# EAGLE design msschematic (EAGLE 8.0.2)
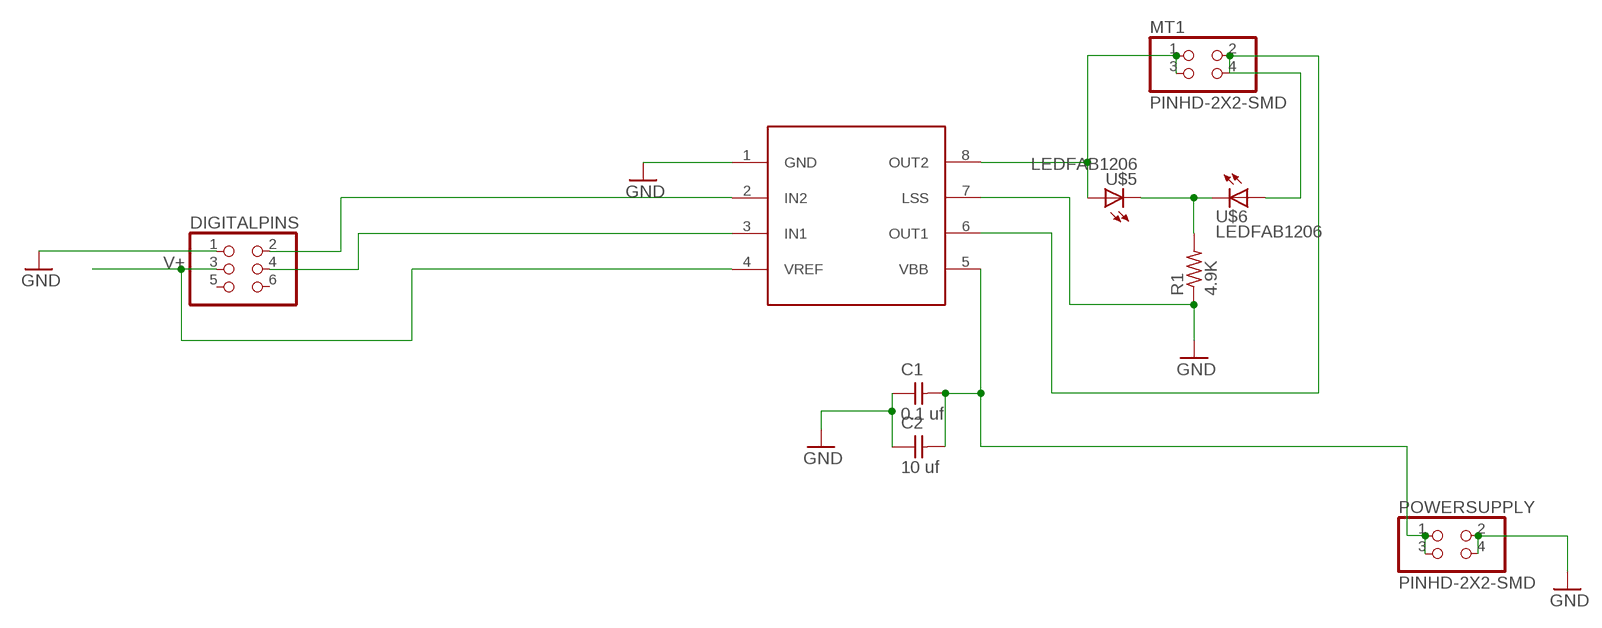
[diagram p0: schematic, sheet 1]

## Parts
C1  0.1 uf  CAP-UNPOLARIZEDFAB  [C1206FAB]
C2  10 uf  CAP-UNPOLARIZEDFAB  [C1206FAB]
DIGITALPINS  PINHD-2X3-SMD  [2X03SMD]
MT1  PINHD-2X2-SMD  [2X02SMD]
POWERSUPPLY  PINHD-2X2-SMD  [2X02SMD]
R1  4.9K  RES-US1206FAB  [R1206FAB]
U$1  A4953-H-BRIDGE-MOTOR-DRIVER  [SOIC8]
U$5  LEDFAB1206  [LED1206FAB]
U$6  LEDFAB1206  [LED1206FAB]

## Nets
GND: C1.1 C2.1 DIGITALPINS.1 POWERSUPPLY.2 POWERSUPPLY.4 R1.1 U$1.1(GND) U$1.7(LSS)
N$1: R1.2 U$5.2(C) U$6.2(C)
N$3: MT1.1 MT1.3 U$1.8(OUT2) U$5.1(A)
N$4: MT1.2 MT1.4 U$1.6(OUT1) U$6.1(A)
N$11: C1.2 C2.2 POWERSUPPLY.1 POWERSUPPLY.3 U$1.5(VBB)
N$16: DIGITALPINS.4 U$1.3(IN1)
N$17: DIGITALPINS.2 U$1.2(IN2)
V+: DIGITALPINS.3 U$1.4(VREF)
Unconnected: DIGITALPINS.5 DIGITALPINS.6

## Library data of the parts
C1 C2 = fab:CAP-UNPOLARIZED
DIGITALPINS = fab:PINHD-2X3-SMD: PIN HEADER
MT1 POWERSUPPLY = fab:PINHD-2X2-SMD
R1 = fab:RES-US: Resistor (US Symbol)
U$1 = fab:A4953-H-BRIDGE-MOTOR-DRIVER
U$5 U$6 = fab:LED: LED

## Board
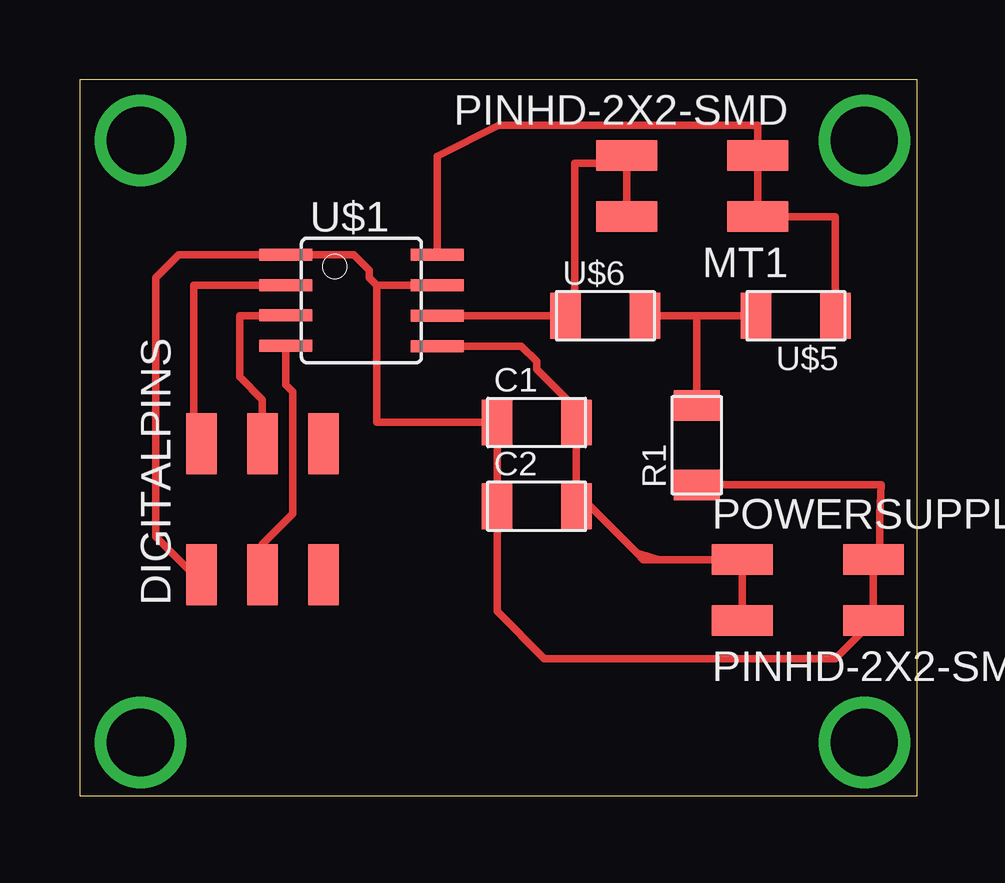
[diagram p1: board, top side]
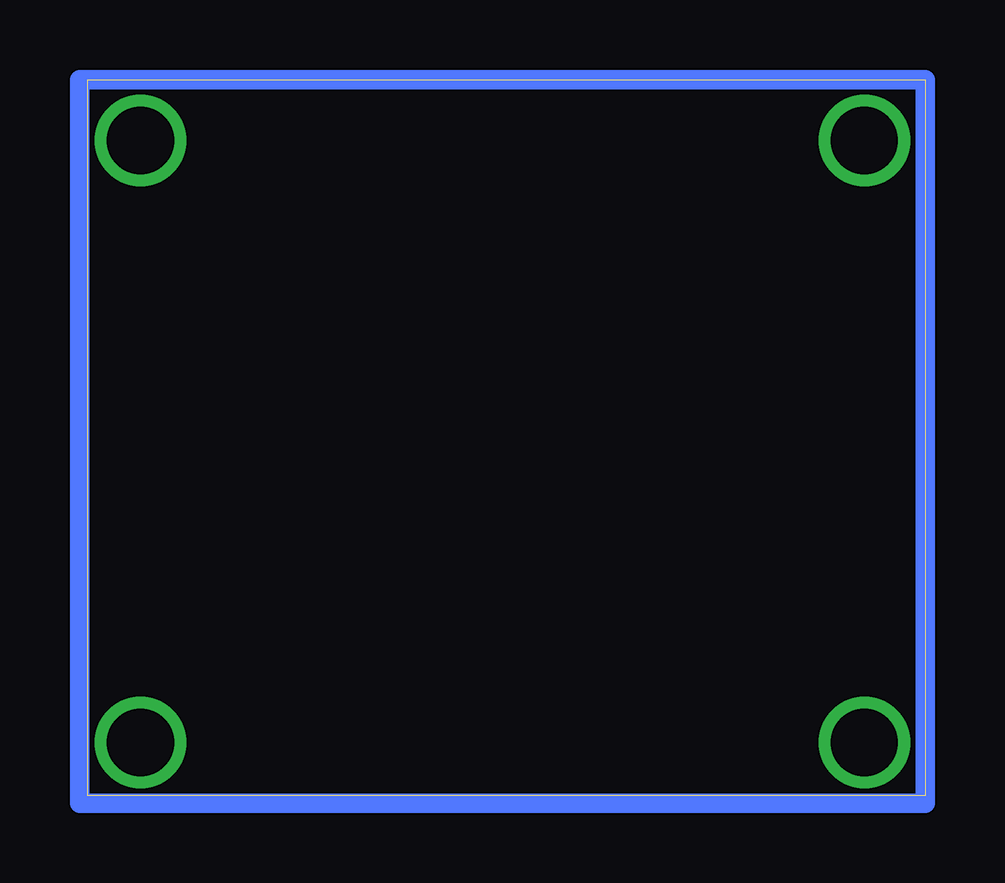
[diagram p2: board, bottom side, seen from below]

Size 34.91 x 29.83 mm. Coordinates in mm from the lower left corner, seen from the top.
Outline: 0,0 34.9,0 34.9,29.83 0,29.83 0,0
Copper layers (1*16): Top 0.035mm / dielectric 1.5mm / Bottom 0.035mm
Design rules "default": minimum track width 10mil, minimum drill 24mil, track to track 8mil, track to pad 8mil, pad to pad 8mil, via to via 8mil, smd to smd 8mil, copper to edge 40mil, drill to drill 8mil, minimum pad ring 10mil, minimum via ring 8mil, stop-mask expansion 4mil, vias tented up to drill 0mil, thermal gap 10mil

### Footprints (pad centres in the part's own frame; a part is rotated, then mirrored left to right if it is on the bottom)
C1206FAB = smd 1.27 x 1.905: 1 -1.651,0; 2 1.651,0
2X03SMD = smd 2.54 x 1.27: 1 -2.54,2.54; 2 2.92,2.54; 3 -2.54,0; 4 2.92,0; 5 -2.54,-2.54; 6 2.92,-2.54
2X02SMD = smd 2.54 x 1.27: 1 -2.54,1.27; 2 2.92,1.27; 3 -2.54,-1.27; 4 2.92,-1.27
R1206FAB = smd 1.27 x 1.905: 1 -1.651,0; 2 1.651,0
SOIC8 = smd 0.5 x 2.2: 1 -1.905,-3.154; 2 -0.645,-3.154; 3 0.625,-3.154; 4 1.895,-3.154; 5 1.905,3.154; 6 0.635,3.154; 7 -0.635,3.154; 8 -1.905,3.154
LED1206FAB = smd 1.27 x 1.905: 1 -1.651,0; 2 1.651,0

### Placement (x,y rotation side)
C1  19.05,15.56 0 top
C2  19.05,12.07 0 top
DIGITALPINS  7.62,11.75 90 top
MT1  25.72,25.4 180 top
POWERSUPPLY  30.16,8.57 0 top
R1  25.72,14.61 90 top
U$1  11.75,20.64 270 top
U$5  29.85,20 180 top
U$6  21.91,20 0 top

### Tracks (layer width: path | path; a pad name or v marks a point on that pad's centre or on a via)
GND
  Top 0.305: 12.38,21.27 12.07,21.59 12.07,21.91 11.43,22.54 U$1.1 4.13,22.54 3.18,21.59 3.18,10.8 4.76,9.21 DIGITALPINS.1 | 15.24,21.27 12.38,21.27 | 15.24,21.27 15.56,21.27 | R1.1 33.4,12.95 33.34,11.75 33.34,10.22 | 33.34,9.84 33.34,10.22 | 33.34,10.22 POWERSUPPLY.2 POWERSUPPLY.4 31.49,5.72 19.37,5.72 17.4,7.68 C2.1 C1.1 12.38,15.56 12.38,21.27 | U$1.7 15.24,21.27
N$1
  Top 0.305: 25.72,20 U$6.2 | 25.72,20 U$5.2 | R1.2 25.72,20
N$3
  Top 0.305: U$5.1 31.5,24.13 MT1.1 MT1.3 28.26,27.94 17.46,27.94 14.9,26.65 U$1.8
N$4
  Top 0.305: MT1.4 MT1.2 22.8,26.35 20.64,26.35 20.64,20 U$6.1 U$1.6
N$8
  Bottom 0.813: 0,29.84 35.24,29.84 35.24,-0.32 0,-0.32 0,29.84
N$11
  Top 0.305: POWERSUPPLY.3 POWERSUPPLY.1 24.13,9.84 | 24.13,9.84 23.49,9.84 23.24,10.1 | 23.24,10.1 21.27,12.07 C2.2 C1.2 20.64,15.62 20.64,16.19 19.05,17.78 19.05,18.1 18.42,18.73 U$1.5 | 23.24,10.1 24.13,9.84
N$12  (via drill 2.8)
  other vias: 2.54,27.3
N$13  (via drill 2.8)
  other vias: 32.7,27.3
N$15  (via drill 2.8)
  other vias: 2.54,2.22
N$16
  Top 0.305: U$1.3 8.59,20 6.67,20 6.67,17.46 7.62,16.51 DIGITALPINS.4
N$17
  Top 0.305: U$1.2 8.59,21.27 4.76,21.27 4.76,14.29 5.08,13.97 DIGITALPINS.2
N$18  (via drill 2.8)
  other vias: 32.7,2.22
V+
  Top 0.305: 7.94,18.74 U$1.4 8.59,17.12 8.89,16.83 8.89,11.75 7.62,10.48 DIGITALPINS.3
